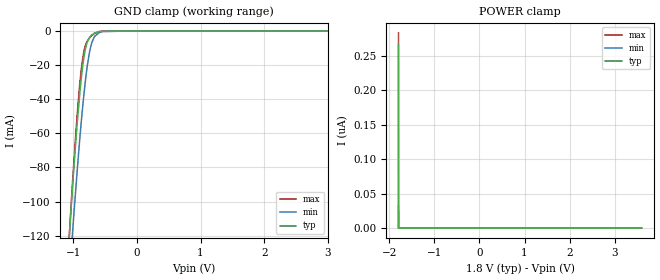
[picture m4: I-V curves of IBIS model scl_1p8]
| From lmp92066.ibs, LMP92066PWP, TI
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|   scl_1p8 Model
[Model]   scl_1p8
Model_type   Input
Vinl = 0.54
Vinh = 1.26
|   typ   min   max
|   (nom PVT)   (fast PVT)   (slow PVT)
C_comp   4.036e-13   3.801e-13   4.850e-13
[Model spec]
|subparameter
Vinl   0.54   0.513   0.567
Vinh   1.26   1.197   1.323
| Where nom  PVT is Nominal Process, 1.8V, 25C
|   Fast PVT is Strong Process,  1.89V, -25C
|   Slow PVT is Weak Process,   1.71V, 125C
[Voltage Range]   1.8   1.71   1.89
|Junction Temperature
[Temperature Range]   25   125   -25
[Power Clamp Reference]   1.8   1.71   1.89
[GND Clamp Reference]   0   0   0
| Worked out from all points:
|   GND clamp passes 1 mA (typ) near -0.65 V on its own axis
[GND Clamp]
|   Voltage   I(typ)   I(min)   I(max)
-1.8V     -632.4mA   -572.3mA   -659.4mA
-1.084V   -133.2mA   -156.2mA   -134.2mA
-1.01V    -90.88mA   -117.9mA   -88.47mA
-926.8mV  -49.46mA   -77.11mA   -44.27mA
-887.4mV  -33.12mA   -59.37mA   -27.69mA
-849.6mV  -20.27mA   -43.92mA   -15.86mA
-798.3mV  -8.92mA    -26.06mA   -7.443mA
-745.4mV  -3.904mA   -12.68mA   -4.035mA
-669.8mV  -1.322mA   -3.483mA   -1.489mA
-539.7mV  -91.43uA   -323.2uA   -92.9uA
-180mV    0A         0A         0A
3.6V      0A         0A         0A
[POWER Clamp]
|   Voltage   I(typ)   I(min)   I(max)
-1.8V     265.5nA    32.44nA    283nA
-1.798V   13.28nA    16.22nA    26.96nA
-1.798V   0A         15.37nA    13.48nA
-1.798V   0A         14.51nA    0A
-1.797V   0A         0A         0A
3.6V      0A         0A         0A
